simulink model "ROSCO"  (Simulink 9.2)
settings: Solver=VariableStepAuto  StartTime=0.0  StopTime=TMax  RelTol=1e-3
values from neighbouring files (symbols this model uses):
  OutList = [OutList    [runFAST.m]    (also in ROSCO2Matlab.m = [])
undefined symbols (not defined in the file or in its folder): cosd, DiscIntNeverNeededParam, F, Parameter, R, rpm2radps, simu, sind, strmatch
libraries: simulink x10
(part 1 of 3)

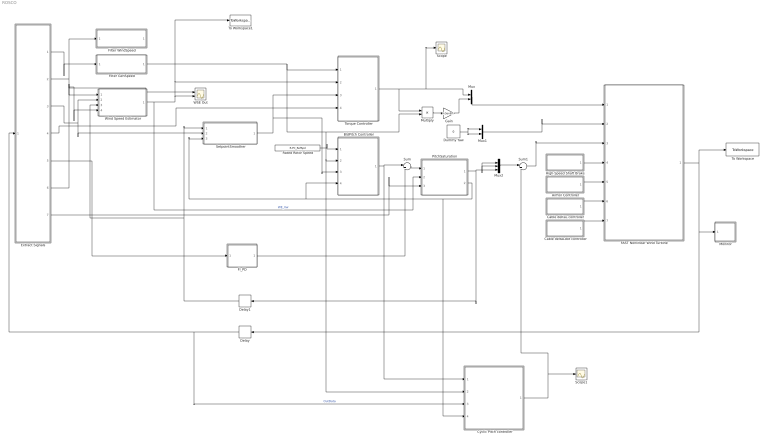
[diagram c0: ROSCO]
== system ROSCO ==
  AirFoil Controller : Subsystem
  BldPitch Controller : Subsystem
  Cable deltaL controller : Subsystem
  Cable deltaLdot controller : Subsystem
  Cyclic Pitch controller : Subsystem  TreatAsAtomicUnit=on
  Delay : Delay  Commented=through  DelayLength=1
  Delay1 : Delay  DelayLength=1
  Dummy Yaw : Constant  Value=0
  Extract Signals : Subsystem  TreatAsAtomicUnit=on
  FAST Nonlinear Wind Turbine : Subsystem
  Filter GenSpeed : Subsystem
  Filter WindSpeed : Subsystem
  Fl_PD : Subsystem
  Gain : Gain  Gain=R.GenEff
  High-Speed Shaft Brake : Subsystem
  Monitor : Subsystem  TreatAsAtomicUnit=on
  Multiply : Product
  Mux : Mux  Inputs=2
  Mux1 : Mux  Inputs=2
  Mux2 : Mux  Inputs=3
  PitchSaturation : Subsystem
  Rated Rotor Speed : Constant  Value=R.PC_RefSpd
  Scope : Scope
  Scope1 : Scope
  SetpointSmoother : Subsystem
  Sum : Sum  Inputs=|++
  Sum1 : Sum  Inputs=|++
  To Workspace : ToWorkspace  VariableName=FAST_Out  SaveFormat=Timeseries  SampleTime=-1
  To Workspace1 : ToWorkspace  VariableName=vhat  SaveFormat=Timeseries  SampleTime=-1
  Torque Controller : Subsystem
  WSE Out : Scope  NumInputPorts=2
  Wind Speed Estimator : Subsystem
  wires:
  FAST Nonlinear Wind Turbine/1(OutData) -> To Workspace/1, Delay/1, Monitor/1(OutData)
  Dummy Yaw/1 -> Mux1/2, Mux1/1
  Mux1/1 -> FAST Nonlinear Wind Turbine/2(Yaw Position (rad) and Rate (rad/s))
  Multiply/1 -> Gain/1
  Extract Signals/1(GenSpeed_rad/s) -> Filter GenSpeed/1(GenSpeed)
  Torque Controller/1(GenTq) -> Scope/1, Mux/1, Multiply/1
  Extract Signals/3(GenTq) -> Wind Speed Estimator/2(tau_g), SetpointSmoother/2(GenTq)
  SetpointSmoother/1(Del_Omega_g) -> BldPitch Controller/3(Del_omega_g), Torque Controller/3(Del_omega_g)
  Rated Rotor Speed/1 -> BldPitch Controller/1(omega_g,ref)
  Gain/1 -> Mux/2
  Extract Signals/2(RtVAvgxh) -> Wind Speed Estimator/4(HorWindV), WSE Out/1, Filter WindSpeed/1(WindSpeed)
  Wind Speed Estimator/1(v_hat) -> PitchSaturation/2(WE_Vw), WSE Out/2, Torque Controller/2(WindSpeedEst), To Workspace1/1  "WE_Vw"
  Delay/1 -> Cyclic Pitch controller/3(OutData), Extract Signals/1(OutData)  "OutData"
  Extract Signals/5(NcIMUTAys) -> Fl_PD/1(NacIMU)
  Fl_PD/1(Fl_Pitcom) -> Sum/2
  Extract Signals/4(BldPitch1) -> Torque Controller/4(BldPitch1)
  Sum/1 -> PitchSaturation/1(PitCom)
  PitchSaturation/1(PitCom_Sat) -> Delay1/1, Mux2/3, Mux2/1, Mux2/2
  PitchSaturation/2(PC_MinPitch) -> Cyclic Pitch controller/4(Min PItch (rad)), BldPitch Controller/4(Min Pitch), SetpointSmoother/3(MinPitch)
  BldPitch Controller/1(BldPitch) -> Cyclic Pitch controller/1(Coll. Pitch), Sum/1
  Extract Signals/6(RotSpeed (rad/s)) -> Wind Speed Estimator/1(omega_r)
  Delay1/1 -> SetpointSmoother/1(BldPitch1), Wind Speed Estimator/3(PitComT)
  Extract Signals/7(TwrFA Accel) -> PitchSaturation/3(TwrFA_Accel)
  Mux/1 -> FAST Nonlinear Wind Turbine/1(Gen. Torque (Nm) and Power (W))
  Filter GenSpeed/1(GenSpeedF) -> Torque Controller/1(GenSpeedF), Multiply/2, BldPitch Controller/2(GenSpeedF), Cyclic Pitch controller/2(Gen Speed)
  Cyclic Pitch controller/1(IPC Cmd (rad,3)) -> Scope1/1, Sum1/2
  Mux2/1 -> Sum1/1
  Sum1/1 -> FAST Nonlinear Wind Turbine/3(Blade Pitch Angles (rad))
  High-Speed Shaft Brake/1(Out1) -> FAST Nonlinear Wind Turbine/4(High-Speed Shaft Braking Fraction (-))
  AirFoil Controller/1(Out1) -> FAST Nonlinear Wind Turbine/5(AirFoil command (-))
  Cable deltaL controller/1(Out1) -> FAST Nonlinear Wind Turbine/6(Cable deltaL command (m))
  Cable deltaLdot controller/1(Out1) -> FAST Nonlinear Wind Turbine/7(Cable deltaLdot command (m/s))

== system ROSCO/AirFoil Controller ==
  Airfoil command : Constant  Value=zeros(1,3)'
  Out1 : Outport  VectorParamsAs1DForOutWhenUnconnected=on
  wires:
  Airfoil command/1 -> Out1/1

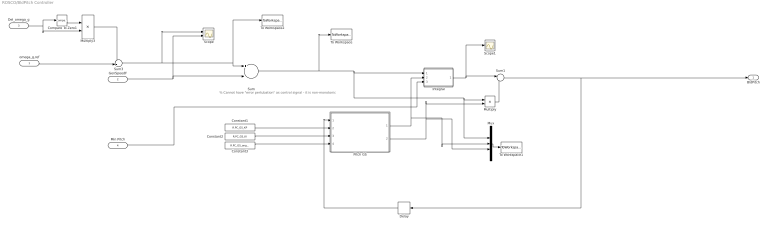
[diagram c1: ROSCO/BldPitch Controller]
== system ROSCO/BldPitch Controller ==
  note: % Cannot have "error pertubation" as control signal - it is non-monotonic
  omega_g,ref : Inport
  GenSpeedF : Inport  Port=2
  Del_omega_g : Inport  Port=3
  Min Pitch : Inport  Port=4
  Compare To Zero1 : simulink/Logic and Bit Operations/Compare To Zero  relop=<  OutDataTypeStr=boolean
  Constant1 : Constant  Value=R.PC_GS_KP
  Constant2 : Constant  Value=R.PC_GS_KI
  Constant3 : Constant  Value=R.PC_GS_angles
  Delay : Delay  DelayLength=1
  Integral : Subsystem
  Multiply : Product
  Multiply3 : Product
  Mux : Mux  Inputs=5
  Pitch GS : MATLAB Function  TreatAsAtomicUnit=on
  Scope : Scope  NumInputPorts=2
  Scope1 : Scope
  Sum : Sum  Inputs=+-
  Sum1 : Sum  Inputs=|++
  Sum3 : Sum  Inputs=-+|
  To Workspace : ToWorkspace  VariableName=SpdErr  SaveFormat=Timeseries  SampleTime=-1
  To Workspace1 : ToWorkspace  VariableName=PC_params  SaveFormat=Structure  SampleTime=-1
  To Workspace2 : ToWorkspace  VariableName=Omega_bg_ref  SaveFormat=Timeseries  SampleTime=-1
  BldPitch : Outport
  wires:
  Multiply/1 -> Sum1/2
  Integral/1(IntSpdErr) -> Scope1/1, Sum1/1
  Pitch GS/1(Ki) -> Mux/3, Integral/2(Gain)
  Pitch GS/2(Kp) -> Mux/4, Multiply/2
  Mux/1 -> To Workspace1/1
  Sum1/1 -> Delay/1, BldPitch/1
  Sum3/1 -> Scope/1, To Workspace2/1, Sum/1
  GenSpeedF/1 -> Scope/2, Sum/2
  Compare To Zero1/1 -> Multiply3/1
  Del_omega_g/1 -> Compare To Zero1/1, Multiply3/2
  Multiply3/1 -> Sum3/1
  omega_g,ref/1 -> Sum3/2
  Constant1/1 -> Pitch GS/2(Kp_pc)
  Constant2/1 -> Pitch GS/3(Ki_pc)
  Constant3/1 -> Pitch GS/4(PC_beta)
  Delay/1 -> Pitch GS/1(Beta)
  Min Pitch/1 -> Integral/3(Min Pitch)
  Sum/1 -> To Workspace/1, Mux/2, Multiply/1, Integral/1(SpeedErr)

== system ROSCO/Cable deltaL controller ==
  Cable deltaL command : Constant  Value=zeros(1,20)'
  Out1 : Outport  VectorParamsAs1DForOutWhenUnconnected=on
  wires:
  Cable deltaL command/1 -> Out1/1

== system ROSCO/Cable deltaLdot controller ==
  Cable deltaLdot command : Constant  Value=zeros(1,20)'
  Out1 : Outport  VectorParamsAs1DForOutWhenUnconnected=on
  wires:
  Cable deltaLdot command/1 -> Out1/1

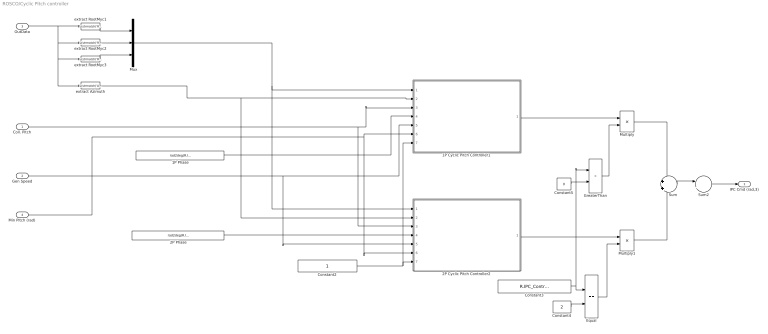
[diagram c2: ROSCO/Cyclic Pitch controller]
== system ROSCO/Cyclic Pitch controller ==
  Coll. Pitch : Inport
  Gen Speed : Inport  Port=2
  OutData : Inport  Port=3
  Min PItch (rad) : Inport  Port=4
  1P Cyclic Pitch Controller1 : Subsystem
  1P Phase : Constant  Value=rad2deg(R.IPC_aziOffset_1P)
  2P Cyclic Pitch Controller2 : Subsystem
  2P Phase : Constant  Value=rad2deg(R.IPC_aziOffset_2P)
  Constant2 : Constant
  Constant3 : Constant  Value=R.IPC_ControlMode
  Constant4 : Constant  Value=2
  Constant5 : Constant  Value=0
  Equal : RelationalOperator  Operator===  OutDataTypeStr=boolean  RndMeth=Simplest
  GreaterThan : RelationalOperator  Operator=>  OutDataTypeStr=boolean  RndMeth=Simplest
  Multiply : Product
  Multiply1 : Product
  Mux : Mux  Inputs=3
  Sum : Sum  Inputs=+|+
  Sum2 : Sum  Inputs=|++
  extract Azimuth : Fcn  Expr=u(strmatch('Azimuth',OutList))
  extract RootMyc1 : Fcn  Expr=u(strmatch('RootMyc1',OutList))
  extract RootMyc2 : Fcn  Expr=u(strmatch('RootMyc2',OutList))
  extract RootMyc3 : Fcn  Expr=u(strmatch('RootMyc3',OutList))
  IPC Cmd (rad,3) : Outport
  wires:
  1P Phase/1 -> 1P Cyclic Pitch Controller1/4(Phase (deg))
  Coll. Pitch/1 -> 2P Cyclic Pitch Controller2/3(Col. Pitch (rad)), 1P Cyclic Pitch Controller1/3(Col. Pitch (rad))
  Gen Speed/1 -> 2P Cyclic Pitch Controller2/5(Gen Speed (rpm)), 1P Cyclic Pitch Controller1/5(Gen Speed (rpm))
  1P Cyclic Pitch Controller1/1(IPC Cmd (rad,3)) -> Multiply/1
  extract RootMyc1/1 -> Mux/1
  extract RootMyc2/1 -> Mux/2
  extract RootMyc3/1 -> Mux/3
  Mux/1 -> 1P Cyclic Pitch Controller1/1(RootMyb), 2P Cyclic Pitch Controller2/1(RootMyb)
  extract Azimuth/1 -> 2P Cyclic Pitch Controller2/2(Azimuth (deg)), 1P Cyclic Pitch Controller1/2(Azimuth (deg))
  Min PItch (rad)/1 -> 2P Cyclic Pitch Controller2/6(Min Pitch (rad)), 1P Cyclic Pitch Controller1/6(Min Pitch (rad))
  2P Phase/1 -> 2P Cyclic Pitch Controller2/4(Phase (deg))
  2P Cyclic Pitch Controller2/1(IPC Cmd (rad,3)) -> Multiply1/1
  Multiply1/1 -> Sum/2
  Multiply/1 -> Sum/1
  OutData/1 -> extract Azimuth/1, extract RootMyc3/1, extract RootMyc2/1, extract RootMyc1/1
  Sum/1 -> Sum2/1
  Sum2/1 -> IPC Cmd (rad,3)/1
  Constant2/1 -> 1P Cyclic Pitch Controller1/7(Enable (-)), 2P Cyclic Pitch Controller2/7(Enable (-))
  Constant4/1 -> Equal/2
  Equal/1 -> Multiply1/2
  Constant3/1 -> GreaterThan/1, Equal/1
  Constant5/1 -> GreaterThan/2
  GreaterThan/1 -> Multiply/2

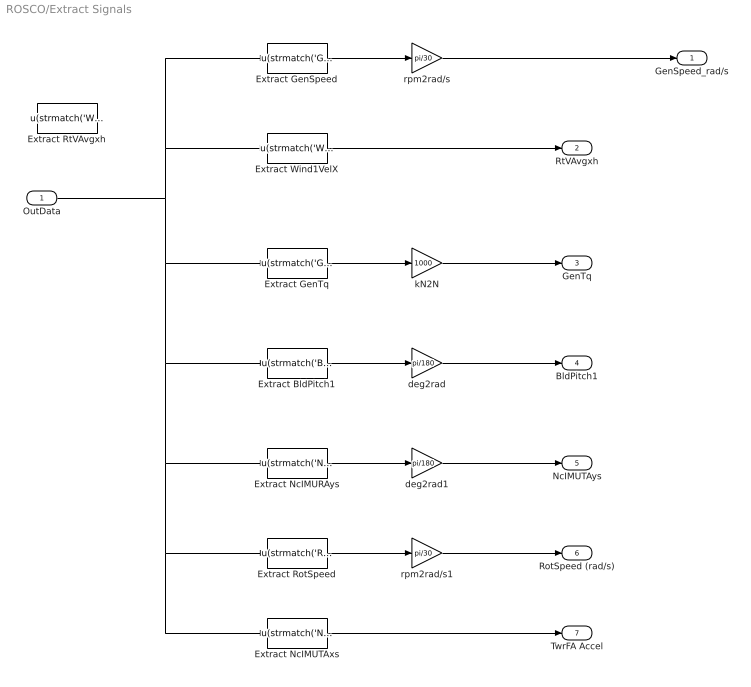
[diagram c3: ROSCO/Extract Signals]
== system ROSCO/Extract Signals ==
  OutData : Inport
  Extract BldPitch1 : Fcn  Expr=u(strmatch('BldPitch1',OutList))
  Extract GenSpeed : Fcn  Expr=u(strmatch('GenSpeed',OutList))
  Extract GenTq : Fcn  Expr=u(strmatch('GenTq',OutList))
  Extract NcIMURAys : Fcn  Expr=u(strmatch('NcIMURAys',OutList))
  Extract NcIMUTAxs : Fcn  Expr=u(strmatch('NcIMUTAxs',OutList))
  Extract RotSpeed : Fcn  Expr=u(strmatch('RotSpeed',OutList))
  Extract RtVAvgxh : Fcn  Commented=on  Expr=u(strmatch('Wind1VelX',OutList))
  Extract Wind1VelX : Fcn  Expr=u(strmatch('Wind1VelX',OutList))
  deg2rad : Gain  Gain=pi/180
  deg2rad1 : Gain  Gain=pi/180
  kN2N : Gain  Gain=1000
  rpm2rad/s : Gain  Gain=pi/30
  rpm2rad/s1 : Gain  Gain=pi/30
  GenSpeed_rad/s : Outport
  RtVAvgxh : Outport  Port=2
  GenTq : Outport  Port=3
  BldPitch1 : Outport  Port=4
  NcIMUTAys : Outport  Port=5
  RotSpeed (rad/s) : Outport  Port=6
  TwrFA Accel : Outport  Port=7
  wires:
  OutData/1 -> Extract Wind1VelX/1, Extract GenSpeed/1, Extract NcIMUTAxs/1, Extract RotSpeed/1, Extract NcIMURAys/1, Extract BldPitch1/1, Extract GenTq/1
  Extract Wind1VelX/1 -> RtVAvgxh/1
  Extract GenSpeed/1 -> rpm2rad/s/1
  Extract BldPitch1/1 -> deg2rad/1
  deg2rad/1 -> BldPitch1/1
  Extract GenTq/1 -> kN2N/1
  kN2N/1 -> GenTq/1
  Extract NcIMURAys/1 -> deg2rad1/1
  deg2rad1/1 -> NcIMUTAys/1
  Extract RotSpeed/1 -> rpm2rad/s1/1
  rpm2rad/s1/1 -> RotSpeed (rad/s)/1
  Extract NcIMUTAxs/1 -> TwrFA Accel/1
  rpm2rad/s/1 -> GenSpeed_rad/s/1

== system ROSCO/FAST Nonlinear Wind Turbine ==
  Gen. Torque (Nm) and Power (W) : Inport
  Yaw Position (rad) and Rate (rad/s) : Inport  Port=2
  Blade Pitch Angles (rad) : Inport  Port=3
  High-Speed Shaft Braking Fraction (-) : Inport  Port=4
  AirFoil command (-) : Inport  Port=5
  Cable deltaL command (m) : Inport  Port=6
  Cable deltaLdot command (m/s) : Inport  Port=7
  Mux1 : Mux  Inputs=7
  S-Function : S-Function  FunctionName=FAST_SFunc  Parameters=FAST_InputFileName, TMax, 43  SFunctionDeploymentMode=off  EnableBusSupport=off
  Signal Specification1 : SignalSpecification  OutDataTypeStr=double  Dimensions=2
  Signal Specification2 : SignalSpecification  OutDataTypeStr=double  Dimensions=2
  OutData : Outport  VectorParamsAs1DForOutWhenUnconnected=on
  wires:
  Gen. Torque (Nm) and Power (W)/1 -> Signal Specification1/1
  S-Function/1 -> OutData/1
  Mux1/1 -> S-Function/1
  Blade Pitch Angles (rad)/1 -> Mux1/3
  Yaw Position (rad) and Rate (rad/s)/1 -> Signal Specification2/1
  Signal Specification1/1 -> Mux1/1
  Signal Specification2/1 -> Mux1/2
  High-Speed Shaft Braking Fraction (-)/1 -> Mux1/4
  AirFoil command (-)/1 -> Mux1/5
  Cable deltaL command (m)/1 -> Mux1/6
  Cable deltaLdot command (m/s)/1 -> Mux1/7

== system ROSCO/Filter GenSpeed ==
  GenSpeed : Inport
  Discrete Filter : DiscreteFilter  Numerator=F.HSS.b  Denominator=F.HSS.a  InitialStates=R.VS_RefSpd/(sum(F.HSS.a(2:end))+1)
  Scope : Scope  NumInputPorts=2
  To Workspace2 : ToWorkspace  VariableName=Om_f  SaveFormat=Timeseries  SampleTime=-1
  GenSpeedF : Outport
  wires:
  Discrete Filter/1 -> Scope/2, To Workspace2/1, GenSpeedF/1
  GenSpeed/1 -> Scope/1, Discrete Filter/1

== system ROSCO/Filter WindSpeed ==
  WindSpeed : Inport
  Discrete Filter : DiscreteFilter  Numerator=F.Wind.b  Denominator=F.Wind.a  InitialStates=10
  To Workspace2 : ToWorkspace  VariableName=WindSpeedF  SaveFormat=Timeseries  SampleTime=-1
  WindSpeedF : Outport
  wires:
  Discrete Filter/1 -> WindSpeedF/1, To Workspace2/1
  WindSpeed/1 -> Discrete Filter/1

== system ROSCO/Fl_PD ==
  NacIMU : Inport
  Constant : Constant
  Enable : Gain  Gain=R.Fl_Mode
  Fl_HPF : DiscreteFilter  Numerator=F.F_Fl_HPF.b  Denominator=F.F_Fl_HPF.b
  Fl_LPF : DiscreteFilter  Numerator=F.F_Fl.b  Denominator=F.F_Fl.a
  Gain1 : Gain  Gain=-R.Fl_Kp
  Integral : Subsystem
  Scope : Scope
  Fl_Pitcom : Outport  VectorParamsAs1DForOutWhenUnconnected=on
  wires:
  Constant/1 -> Integral/2(Gain)
  NacIMU/1 -> Fl_LPF/1  "FA_AccR"
  Integral/1(Int x) -> Gain1/1
  Fl_HPF/1 -> Integral/1(x)  "FA_AccF"
  Gain1/1 -> Enable/1  "Fl_Pitcom"
  Enable/1 -> Scope/1, Fl_Pitcom/1  "Fl_Pitcom"
  Fl_LPF/1 -> Fl_HPF/1  "FA_AccF"

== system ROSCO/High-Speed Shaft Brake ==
  High-Speed Shaft Braking Fraction : Constant  Value=0
  Out1 : Outport  VectorParamsAs1DForOutWhenUnconnected=on
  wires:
  High-Speed Shaft Braking Fraction/1 -> Out1/1

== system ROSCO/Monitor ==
  OutData : Inport
  Extract BldPitch1 : Fcn  Expr=u(strmatch('BldPitch1',OutList))
  Extract GenTq : Fcn  Expr=u(strmatch('GenTq',OutList))
  Extract RotSpeed : Fcn  Expr=u(strmatch('RotSpeed',OutList))
  Scope : Scope  NumInputPorts=3
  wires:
  Extract BldPitch1/1 -> Scope/3
  OutData/1 -> Extract RotSpeed/1, Extract BldPitch1/1, Extract GenTq/1
  Extract RotSpeed/1 -> Scope/1
  Extract GenTq/1 -> Scope/2

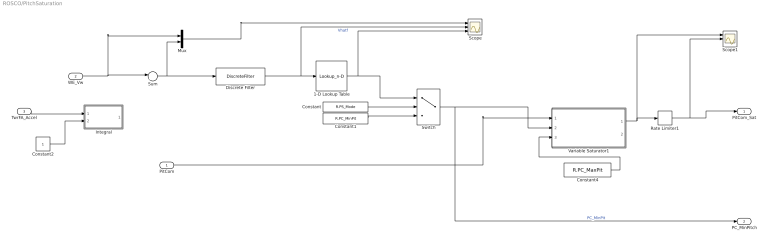
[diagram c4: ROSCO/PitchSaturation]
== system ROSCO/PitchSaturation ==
  PitCom : Inport
  WE_Vw : Inport  Port=2
  TwrFA_Accel : Inport  Port=3
  1-D Lookup Table : Lookup_n-D  NumberOfTableDimensions=1  BreakpointsForDimension1=R.PS_WindSpeeds  Table=R.PS_BldPitchMin  InternalRulePriority=Speed  RndMeth=Simplest
  Constant : Constant  Value=R.PS_Mode
  Constant1 : Constant  Value=R.PC_MinPit
  Constant2 : Constant
  Constant4 : Constant  Value=R.PC_MaxPit
  Discrete Filter : DiscreteFilter  Numerator=F.F_PS.b  Denominator=F.F_PS.a  InitialStates=R.WE_v0/(sum(F.F_PS.a(2:end))+1)
  Integral : Subsystem
  Mux : Mux  Inputs=2
  Rate Limiter1 : RateLimiter  RisingSlewLimit=R.PC_MaxRat  FallingSlewLimit=-R.PC_MaxRat  SampleTimeMode=inherited
  Scope : Scope  NumInputPorts=3
  Scope1 : Scope  NumInputPorts=3
  Sum : Sum  Inputs=|++
  Switch : Switch  Criteria=u2 > Threshold  Threshold=0.5
  Variable Saturator1 : MATLAB Function  TreatAsAtomicUnit=on
  PitCom_Sat : Outport  VectorParamsAs1DForOutWhenUnconnected=on
  PC_MinPitch : Outport  Port=2  VectorParamsAs1DForOutWhenUnconnected=on
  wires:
  1-D Lookup Table/1 -> Scope/3, Switch/1
  Constant/1 -> Switch/2
  Discrete Filter/1 -> Scope/2, 1-D Lookup Table/1  "Vhatf"
  Constant1/1 -> Switch/3
  Switch/1 -> PC_MinPitch/1, Variable Saturator1/2(lowerLimit)  "PC_MinPit"
  Constant4/1 -> Variable Saturator1/3(upperLimit)
  Variable Saturator1/1(pitchCommandOut) -> Scope1/1, Rate Limiter1/1
  Rate Limiter1/1 -> Scope1/2, PitCom_Sat/1
  PitCom/1 -> Variable Saturator1/1(pitchCommand)
  TwrFA_Accel/1 -> Integral/1(x)
  Constant2/1 -> Integral/2(Gain)
  WE_Vw/1 -> Mux/1, Sum/1
  Sum/1 -> Mux/2, Discrete Filter/1
  Mux/1 -> Scope/1

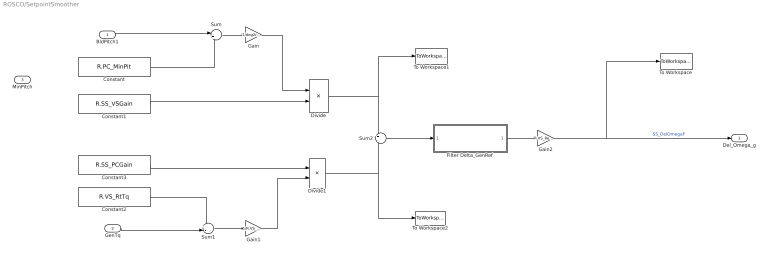
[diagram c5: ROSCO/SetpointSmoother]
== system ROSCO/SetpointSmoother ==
  BldPitch1 : Inport
  GenTq : Inport  Port=2
  MinPitch : Inport  Port=3
  Constant : Constant  Value=R.PC_MinPit
  Constant1 : Constant  Value=R.SS_VSGain
  Constant2 : Constant  Value=R.VS_RtTq
  Constant3 : Constant  Value=R.SS_PCGain
  Divide : Product  Inputs=**
  Divide1 : Product  Inputs=**
  Filter Delta_GenRef : Subsystem
  Gain : Gain  Gain=1/deg2rad(30)
  Gain1 : Gain  Gain=1/R.VS_RtTq
  Gain2 : Gain  Gain=R.VS_RefSpd
  Sum : Sum  Inputs=|+-
  Sum1 : Sum  Inputs=+-|
  Sum2 : Sum  Inputs=+|-
  To Workspace : ToWorkspace  VariableName=DelOmega  SaveFormat=Timeseries  SampleTime=-1
  To Workspace1 : ToWorkspace  VariableName=BldPitch_GB  SaveFormat=Timeseries  SampleTime=-1
  To Workspace2 : ToWorkspace  VariableName=Torque_GB  SaveFormat=Timeseries  SampleTime=-1
  Del_Omega_g : Outport
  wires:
  Divide1/1 -> Sum2/2, To Workspace2/1
  Divide/1 -> Sum2/1, To Workspace1/1
  Filter Delta_GenRef/1(GainBiasF) -> Gain2/1
  Constant3/1 -> Divide1/1
  Constant1/1 -> Divide/2
  Sum/1 -> Gain/1
  BldPitch1/1 -> Sum/1
  Sum2/1 -> Filter Delta_GenRef/1(GainBias)
  Constant2/1 -> Sum1/1
  Sum1/1 -> Gain1/1
  GenTq/1 -> Sum1/2
  Gain/1 -> Divide/1
  Gain1/1 -> Divide1/2
  Gain2/1 -> To Workspace/1, Del_Omega_g/1  "SS_DelOmegaF"
  Constant/1 -> Sum/2

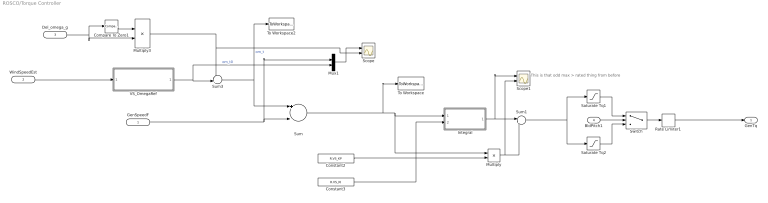
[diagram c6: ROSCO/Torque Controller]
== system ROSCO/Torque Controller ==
  note: This is that odd max > rated thing from before
  GenSpeedF : Inport
  WindSpeedEst : Inport  Port=2
  Del_omega_g : Inport  Port=3
  BldPitch1 : Inport  Port=4
  Compare To Zero1 : simulink/Logic and Bit Operations/Compare To Zero  relop=>  OutDataTypeStr=boolean
  Constant2 : Constant  Value=R.VS_KP
  Constant3 : Constant  Value=R.VS_KI
  Integral : Subsystem
  Multiply : Product
  Multiply3 : Product
  Mux1 : Mux  Inputs=2
  Rate Limiter1 : RateLimiter  RisingSlewLimit=R.VS_MaxRat  FallingSlewLimit=-R.VS_MaxRat  SampleTimeMode=inherited  InitialCondition=R.VS_RtTq
  Saturate Tq1 : Saturate  UpperLimit=R.VS_RtTq  LowerLimit=0
  Saturate Tq2 : Saturate  UpperLimit=R.VS_RtTq  LowerLimit=0
  Scope : Scope  NumInputPorts=2
  Scope1 : Scope  NumInputPorts=2
  Sum : Sum  Inputs=+-
  Sum1 : Sum  Inputs=|++
  Sum3 : Sum  Inputs=-+|
  Switch : Switch  Criteria=u2 > Threshold  Threshold=R.VS_Rgn3MP
  To Workspace : ToWorkspace  VariableName=VSdiff  SaveFormat=Timeseries  SampleTime=-1
  To Workspace2 : ToWorkspace  VariableName=Omega_tg_ref  SaveFormat=Timeseries  SampleTime=-1
  VS_OmegaRef : Subsystem
  GenTq : Outport
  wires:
  Multiply/1 -> Scope1/2, Sum1/2
  Integral/1(IntSpdErr) -> Scope1/1, Sum1/1
  Constant2/1 -> Multiply/2
  Constant3/1 -> Integral/2(Gain)
  VS_OmegaRef/1(VS_OmegaOpt) -> Mux1/2, Sum3/2  "om_t0"
  GenSpeedF/1 -> Mux1/1, Sum/2
  Sum3/1 -> To Workspace2/1, Sum/1  "om_t"
  Saturate Tq2/1 -> Switch/3
  Switch/1 -> Rate Limiter1/1
  Saturate Tq1/1 -> Switch/1
  BldPitch1/1 -> Switch/2
  Compare To Zero1/1 -> Multiply3/1
  Del_omega_g/1 -> Compare To Zero1/1, Multiply3/2
  Multiply3/1 -> Scope/2, Sum3/1
  Mux1/1 -> Scope/1
  Sum1/1 -> Saturate Tq2/1, Saturate Tq1/1
  Rate Limiter1/1 -> GenTq/1
  Sum/1 -> To Workspace/1, Integral/1(SpeedErr), Multiply/1
  WindSpeedEst/1 -> VS_OmegaRef/1(WindSpeedEst)

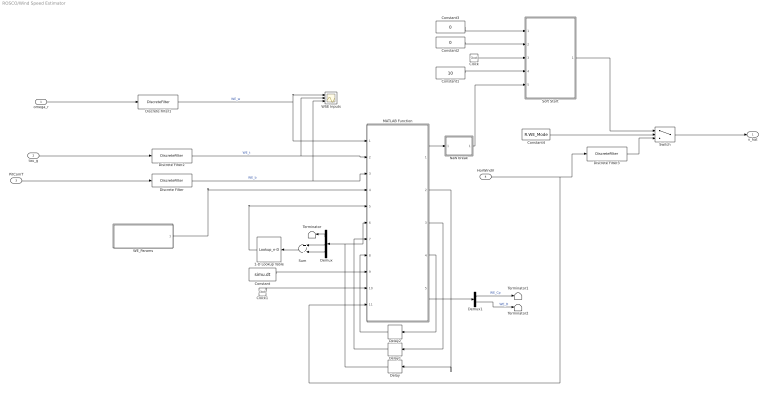
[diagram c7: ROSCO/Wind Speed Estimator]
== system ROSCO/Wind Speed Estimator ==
  omega_r : Inport
  tau_g : Inport  Port=2
  PitComT : Inport  Port=3
  HorWindV : Inport  Port=4
  1-D Lookup Table : Lookup_n-D  NumberOfTableDimensions=1  BreakpointsForDimension1=[-5:5]  Table=tanh([-5:5])  InternalRulePriority=Speed  RndMeth=Simplest
  Clock : Clock
  Clock1 : Clock
  Constant : Constant  Value=simu.dt
  Constant1 : Constant  Value=10
  Constant2 : Constant  Value=0
  Constant3 : Constant  Value=0
  Constant4 : Constant  Value=R.WE_Mode
  Delay : Delay  DelayLength=1  InitialCondition=[R.WE_GearboxRatio, 0, R.WE_v0]'
  Delay1 : Delay  DelayLength=1  InitialCondition=diag([0.1, 0.1, 1])^2
  Delay2 : Delay  DelayLength=1  InitialCondition=zeros(3,1)
  Demux : Demux  Outputs=3
  Demux1 : Demux  Outputs=2
  Discrete Filter : DiscreteFilter  Numerator=F.F_WSEBlPitch.b  Denominator=F.F_WSEBlPitch.a
  Discrete Filter1 : DiscreteFilter  Numerator=F.HSS.b  Denominator=F.HSS.a  InitialStates=R.VS_RefSpd/(sum(F.HSS.a(2:end))+1)/R.GBRatio
  Discrete Filter2 : DiscreteFilter  Numerator=F.F_GenTq.b  Denominator=F.F_GenTq.a  InitialStates=R.VS_RtTq/(sum(F.F_GenTq.a(2:end))+1)
  Discrete Filter3 : DiscreteFilter  Numerator=F.Wind.b  Denominator=F.Wind.a  InitialStates=10
  MATLAB Function : MATLAB Function  TreatAsAtomicUnit=on
  NaN break : MATLAB Function  TreatAsAtomicUnit=on
  Soft Start : MATLAB Function  TreatAsAtomicUnit=on
  Sum : Sum
  Switch : Switch  Criteria=u2 > Threshold  Threshold=0.5
  Terminator : Terminator
  Terminator1 : Terminator
  Terminator2 : Terminator
  WE_Params : Subsystem
  WSE Inputs : Scope  NumInputPorts=3
  v_hat : Outport
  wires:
  MATLAB Function/2(xh) -> Delay/1
  Delay/1 -> Demux/1, MATLAB Function/6("xh ")
  MATLAB Function/3(P) -> Delay1/1
  Delay1/1 -> MATLAB Function/7("P ")
  omega_r/1 -> Discrete Filter1/1
  tau_g/1 -> Discrete Filter2/1
  MATLAB Function/4(K) -> Delay2/1
  Delay2/1 -> MATLAB Function/8("K ")
  Constant/1 -> MATLAB Function/9(dt)
  Demux/2 -> Sum/1
  Demux/3 -> Sum/2
  Demux/1 -> Terminator/1
  Sum/1 -> 1-D Lookup Table/1
  1-D Lookup Table/1 -> MATLAB Function/5(A_op)
  WE_Params/1(WE_Params) -> MATLAB Function/4(WE_params)
  Clock/1 -> Soft Start/3(time)
  Constant1/1 -> Soft Start/4(generic)
  Constant2/1 -> Soft Start/2(endTime)
  Constant3/1 -> Soft Start/1(startTime)
  MATLAB Function/1(vh) -> NaN break/1(u)
  Discrete Filter/1 -> WSE Inputs/3, MATLAB Function/3(beta)  "WE_b"
  Discrete Filter1/1 -> MATLAB Function/1(omega_r), WSE Inputs/1  "WE_w"
  Discrete Filter2/1 -> MATLAB Function/2(tau_g), WSE Inputs/2  "WE_t"
  PitComT/1 -> Discrete Filter/1
  Soft Start/1(out) -> Switch/1
  Switch/1 -> v_hat/1
  HorWindV/1 -> MATLAB Function/11(HorWind), Discrete Filter3/1
  Constant4/1 -> Switch/2
  MATLAB Function/5(Debug) -> Demux1/1
  Demux1/1 -> Terminator1/1  "WE_Cp"
  Demux1/2 -> Terminator2/1  "WE_D"
  Clock1/1 -> MATLAB Function/10(t)
  Discrete Filter3/1 -> Switch/3
  NaN break/1(y) -> Soft Start/5(actual)

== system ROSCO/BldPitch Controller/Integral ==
  SpeedErr : Inport
  Gain : Inport  Port=2
  Min Pitch : Inport  Port=3
  Gain1 : Gain  Gain=simu.dt
  Maximum Pitch : Constant  Value=R.PC_MaxPit
  Minimum Pitch : Constant  Value=R.PC_MinPit
  Multiply : Product
  Saturate Integral Term : simulink/Discontinuities/Saturation Dynamic  OutMin=[]  OutMax=[]  OutDataTypeStr=Inherit: Same as second input  OutDataType=fixdt(1, 16)  OutScaling=2^-10  RndMeth=Nearest  DoSatur=off
  Sum : Sum  Inputs=|++
  Unit Delay : UnitDelay  SampleTime=-1
  IntSpdErr : Outport
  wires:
  Maximum Pitch/1 -> Saturate Integral Term/1
  Unit Delay/1 -> Sum/2
  Sum/1 -> Saturate Integral Term/2
  SpeedErr/1 -> Gain1/1
  Gain/1 -> Multiply/2
  Saturate Integral Term/1 -> IntSpdErr/1, Unit Delay/1
  Gain1/1 -> Multiply/1
  Multiply/1 -> Sum/1
  Min Pitch/1 -> Saturate Integral Term/3

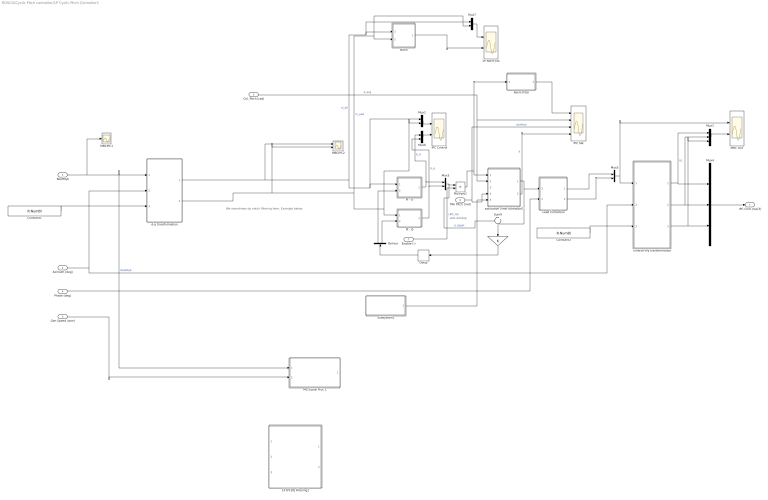
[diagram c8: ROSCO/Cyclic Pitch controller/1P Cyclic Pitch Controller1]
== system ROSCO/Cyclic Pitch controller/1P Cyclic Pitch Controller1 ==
  note: We sometimes do notch filtering here. Example below.
  note: k
  note: anti-windup
  RootMyb : Inport
  Azimuth (deg) : Inport  Port=2
  Col. Pitch (rad) : Inport  Port=3
  Phase (deg) : Inport  Port=4
  Gen Speed (rpm) : Inport  Port=5
  Min Pitch (rad) : Inport  Port=6
  Enable (-) : Inport  Port=7
  " " : Gain
  1P IPCDQ Filtering1 : Subsystem  Commented=on
  1P Norm Est : Scope  NumInputPorts=2
  Constant1 : Constant  Value=R.NumBl
  Constant2 : Constant  Value=R.NumBl
  Delay : Delay  DelayLength=1
  Demux : Demux  Outputs=2
  IPC Control : Scope  NumInputPorts=2
  IPC Sat : Scope  NumInputPorts=4
  Lead Correction : MATLAB Function  TreatAsAtomicUnit=on
  M0 Signal Proc.1 : Subsystem  Commented=on
  MBC Out : Scope  NumInputPorts=2
  MBCIPC1 : Scope
  MBCIPC2 : Scope  NumInputPorts=2
  Multiply1 : Product
  Mux1 : Mux  Inputs=3
  Mux{2..3,5..7} (5 alike) : Mux  Inputs=2
  Mux4 : Mux  Inputs=3
  Norm : Subsystem  Commented=on
  Norm Pitch : Subsystem  Commented=on
  PI - D : Subsystem  TreatAsAtomicUnit=on  SystemSampleTime=simu.dt
  PI - Q : Subsystem  TreatAsAtomicUnit=on  SystemSampleTime=simu.dt
  Subsystem1 : Subsystem
  Sum9 : Sum  Inputs=-|+
  d-q transformation : MATLAB Function  TreatAsAtomicUnit=on
  inverse d-q transformation : MATLAB Function  TreatAsAtomicUnit=on
  saturation (limit schedule)1 : MATLAB Function  TreatAsAtomicUnit=on
  IPC Cmd (rad,3) : Outport
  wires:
  Col. Pitch (rad)/1 -> saturation (limit schedule)1/2(b_avg), IPC Sat/2  "b_avg"
  saturation (limit schedule)1/1(bdq) -> Sum9/2, Lead Correction/1(bdq)
  Gen Speed (rpm)/1 -> M0 Signal Proc.1/2(GenSpeed)
  d-q transformation/1(M_tilt) -> Mux2/1, PI - D/1(Md), Mux7/1, Norm/1(In1), MBCIPC2/1  "m_tilt"
  Mux5/1 -> MBC Out/1, inverse d-q transformation/1(bdq)
  inverse d-q transformation/3(b3) -> Mux1/3, Mux4/3
  Phase (deg)/1 -> Lead Correction/2(psi_o)
  PI - Q/1(Theta_yaw) -> Mux6/2, Mux3/2  "b_q"
  PI - D/1(Theta_tilt) -> Mux3/1, Mux6/1  "b_d"
  Demux/1 -> PI - D/2(Anti-windup)
  inverse d-q transformation/1(b1) -> Mux1/1, Mux4/1  "b1"
  Demux/2 -> PI - Q/2(Anti-windup)
  inverse d-q transformation/2(b2) -> Mux1/2, Mux4/2
  Mux4/1 -> IPC Cmd (rad,3)/1
  Delay/1 -> Demux/1
  " "/1 -> Delay/1
  RootMyb/1 -> M0 Signal Proc.1/1("My1,2, 3"), d-q transformation/1(RootMyb), MBCIPC1/1  "RootMyb"
  Sum9/1 -> " "/1
  Azimuth (deg)/1 -> d-q transformation/2(Az), inverse d-q transformation/2(Az)
  Lead Correction/1(b_cos) -> Mux5/1
  Lead Correction/2(b_sin) -> Mux5/2
  saturation (limit schedule)1/2(k) -> IPC Sat/4
  Constant1/1 -> d-q transformation/3(NumBl)
  Constant2/1 -> inverse d-q transformation/3(NumBl)
  d-q transformation/2(M_yaw) -> Mux2/2, PI - Q/1(Mq), Mux7/2, Norm/2(In2), MBCIPC2/2  "m_yaw"
  Mux1/1 -> MBC Out/2
  Mux6/1 -> IPC Control/2
  Mux2/1 -> IPC Control/1
  Mux7/1 -> 1P Norm Est/1
  Norm/1(Out1) -> 1P Norm Est/2
  Min Pitch (rad)/1 -> IPC Sat/3, saturation (limit schedule)1/4(minPitch)  "minPitch"
  Norm Pitch/1(Out1) -> IPC Sat/1
  Enable (-)/1 -> Multiply1/2  "cIPC_GS"
  Subsystem1/1(IPC Sat Params) -> saturation (limit schedule)1/5(Params)
  Mux3/1 -> Sum9/1, Multiply1/1  "b_dqsat"
  Multiply1/1 -> Norm Pitch/1(b_dqsat), saturation (limit schedule)1/1(bdq_unsat)
  ? -> 1P IPCDQ Filtering1/2(My)  "m_yaw"

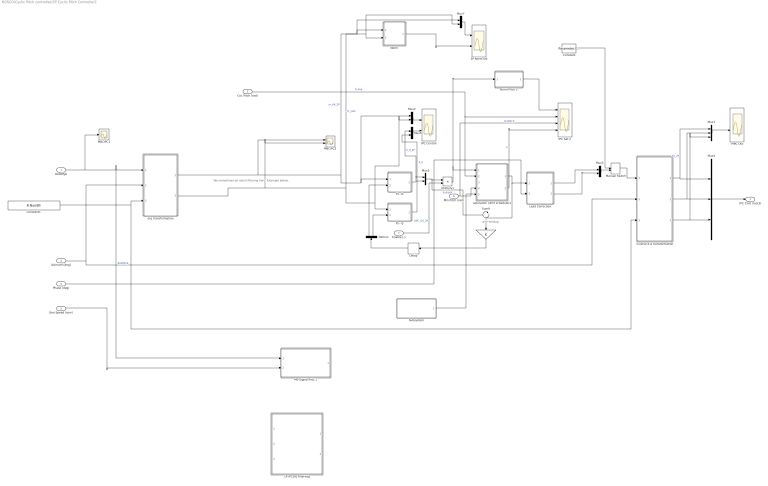
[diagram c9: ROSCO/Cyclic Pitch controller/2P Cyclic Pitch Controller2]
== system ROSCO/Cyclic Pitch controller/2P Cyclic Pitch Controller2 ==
  note: We sometimes do notch filtering here. Example below.
  note: anti-windup
  note: k
  RootMyb : Inport
  Azimuth (deg) : Inport  Port=2
  Col. Pitch (rad) : Inport  Port=3
  Phase (deg) : Inport  Port=4
  Gen Speed (rpm) : Inport  Port=5
  Min Pitch (rad) : Inport  Port=6
  Enable (-) : Inport  Port=7
  " " : Gain
  1P IPCDQ Filtering1 : Subsystem  Commented=on
  2P Norm Est : Scope  NumInputPorts=2
  Constant : Constant  Commented=on  Value=Parameter.Control.cIPC.OL_2P.amp * [cosd(Parameter.Control.cIPC.OL_2P.phase), sind(Parameter.Control.cIPC.OL_2P.phase)]
  Constant1 : Constant  Value=R.NumBl
  Delay : Delay  DelayLength=1
  Demux : Demux  Outputs=2
  IPC Control : Scope  NumInputPorts=2
  IPC Sat 2 : Scope  NumInputPorts=4
  Lead Correction : MATLAB Function  TreatAsAtomicUnit=on
  M0 Signal Proc.1 : Subsystem  Commented=on
  MBC Out : Scope  NumInputPorts=2
  MBCIPC1 : Scope
  MBCIPC2 : Scope  NumInputPorts=2
  Manual Switch : ManualSwitch  CurrentSetting=0
  Multiply1 : Product
  Mux1 : Mux  Inputs=3
  Mux{2..3,5..7} (5 alike) : Mux  Inputs=2
  Mux4 : Mux  Inputs=3
  Norm : Subsystem  Commented=on
  Norm Pitch 2 : Subsystem  Commented=on
  PI - D : Subsystem  TreatAsAtomicUnit=on  SystemSampleTime=simu.dt
  PI - Q : Subsystem  TreatAsAtomicUnit=on  SystemSampleTime=simu.dt
  Subsystem : Subsystem
  Sum9 : Sum  Inputs=-|+
  d-q transformation : MATLAB Function  TreatAsAtomicUnit=on
  inverse d-q transformation : MATLAB Function  TreatAsAtomicUnit=on
  saturation (limit schedule)1 : MATLAB Function  TreatAsAtomicUnit=on
  IPC Cmd (rad,3) : Outport
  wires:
  Enable (-)/1 -> Multiply1/2  "cIPC_GS_2P"
  Norm Pitch 2/1(Out1) -> IPC Sat 2/1
  Min Pitch (rad)/1 -> saturation (limit schedule)1/4(minPitch), IPC Sat 2/3  "minPitch"
  Norm/1(Out1) -> 2P Norm Est/2
  Mux7/1 -> 2P Norm Est/1
  Mux2/1 -> IPC Control/1
  Mux6/1 -> IPC Control/2
  Mux1/1 -> MBC Out/2
  d-q transformation/2(M_yaw) -> PI - Q/1(Mq), Mux2/2, Norm/2(In2), Mux7/2, MBCIPC2/2  "m_yaw"
  Constant1/1 -> inverse d-q transformation/3(NumBl), d-q transformation/3(NumBl)
  saturation (limit schedule)1/2(k) -> IPC Sat 2/4
  Lead Correction/2(b_sin) -> Mux5/2
  Lead Correction/1(b_cos) -> Mux5/1
  Azimuth (deg)/1 -> inverse d-q transformation/2(Az), d-q transformation/2(Az)
  Sum9/1 -> " "/1
  RootMyb/1 -> MBCIPC1/1, M0 Signal Proc.1/1("My1,2, 3"), d-q transformation/1(RootMyb)  "RootMyb"
  " "/1 -> Delay/1
  Delay/1 -> Demux/1
  Mux4/1 -> IPC Cmd (rad,3)/1
  inverse d-q transformation/2(b2) -> Mux4/2, Mux1/2
  Demux/2 -> PI - Q/2(Anti-windup)
  inverse d-q transformation/1(b1) -> Mux4/1, Mux1/1  "b1_2P"
  Demux/1 -> PI - D/2(Anti-windup)
  PI - D/1(Theta_tilt) -> Mux6/1, Mux3/1  "b_d_2P"
  PI - Q/1(Theta_yaw) -> Mux6/2, Mux3/2  "b_q"
  Phase (deg)/1 -> Lead Correction/2(psi_o)
  inverse d-q transformation/3(b3) -> Mux4/3, Mux1/3
  d-q transformation/1(M_tilt) -> PI - D/1(Md), Mux2/1, Norm/1(In1), Mux7/1, MBCIPC2/1  "m_tilt_2P"
  Gen Speed (rpm)/1 -> M0 Signal Proc.1/2(GenSpeed)
  saturation (limit schedule)1/1(bdq) -> Lead Correction/1(bdq), Sum9/2
  Col. Pitch (rad)/1 -> IPC Sat 2/2, saturation (limit schedule)1/2(b_avg)  "b_avg"
  Subsystem/1(IPC Sat Params) -> saturation (limit schedule)1/5(Params)
  Mux3/1 -> Sum9/1, Multiply1/1  "b_dqsat"
  Multiply1/1 -> Norm Pitch 2/1(b_dqsat), saturation (limit schedule)1/1(bdq_unsat)
  Mux5/1 -> Manual Switch/2
  Manual Switch/1 -> inverse d-q transformation/1(bdq)
  Constant/1 -> Manual Switch/1

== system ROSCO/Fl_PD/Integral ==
  x : Inport
  Gain : Inport  Port=2
  Gain1 : Gain  Gain=simu.dt
  Maximum Pitch : Constant  Value=100
  Minimum Pitch : Constant  Value=-100
  Multiply : Product
  Saturate Integral Term : simulink/Discontinuities/Saturation Dynamic  OutMin=[]  OutMax=[]  OutDataTypeStr=Inherit: Same as second input  OutDataType=fixdt(1, 16)  OutScaling=2^-10  RndMeth=Nearest  DoSatur=off
  Scope : Scope  NumInputPorts=2
  Sum : Sum  Inputs=|++
  Unit Delay : UnitDelay  SampleTime=-1
  Int x : Outport
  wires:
  Maximum Pitch/1 -> Saturate Integral Term/1
  Unit Delay/1 -> Sum/2
  Minimum Pitch/1 -> Saturate Integral Term/3
  Sum/1 -> Saturate Integral Term/2
  x/1 -> Scope/1, Gain1/1
  Gain/1 -> Multiply/2
  Saturate Integral Term/1 -> Scope/2, Int x/1, Unit Delay/1
  Gain1/1 -> Multiply/1
  Multiply/1 -> Sum/1

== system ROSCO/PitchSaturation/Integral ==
  x : Inport
  Gain : Inport  Port=2
  Gain1 : Gain  Gain=simu.dt
  Maximum Pitch : Constant  Value=100
  Minimum Pitch : Constant  Value=-100
  Multiply : Product
  Saturate Integral Term : simulink/Discontinuities/Saturation Dynamic  OutMin=[]  OutMax=[]  OutDataTypeStr=Inherit: Same as second input  OutDataType=fixdt(1, 16)  OutScaling=2^-10  RndMeth=Nearest  DoSatur=off
  Scope : Scope  NumInputPorts=2
  Sum : Sum  Inputs=|++
  Unit Delay : UnitDelay  SampleTime=-1
  Int x : Outport
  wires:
  Maximum Pitch/1 -> Saturate Integral Term/1
  Unit Delay/1 -> Sum/2
  Minimum Pitch/1 -> Saturate Integral Term/3
  Sum/1 -> Saturate Integral Term/2
  x/1 -> Scope/1, Gain1/1
  Gain/1 -> Multiply/2
  Saturate Integral Term/1 -> Scope/2, Int x/1, Unit Delay/1
  Gain1/1 -> Multiply/1
  Multiply/1 -> Sum/1

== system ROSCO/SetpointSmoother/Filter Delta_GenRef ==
  GainBias : Inport
  Discrete Filter : DiscreteFilter  Numerator=F.F_SS.b  Denominator=F.F_SS.a
  GainBiasF : Outport
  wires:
  Discrete Filter/1 -> GainBiasF/1
  GainBias/1 -> Discrete Filter/1

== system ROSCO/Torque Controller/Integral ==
  SpeedErr : Inport
  Gain : Inport  Port=2
  Gain1 : Gain  Gain=simu.dt
  Maximum Torque : Constant  Value=R.VS_RtTq
  Minimum Torque : Constant  Value=0
  Multiply : Product
  Saturate Integral Term : simulink/Discontinuities/Saturation Dynamic  OutMin=[]  OutMax=[]  OutDataTypeStr=Inherit: Same as second input  OutDataType=fixdt(1, 16)  OutScaling=2^-10  RndMeth=Nearest  DoSatur=off
  Sum : Sum  Inputs=|++
  Unit Delay : UnitDelay  InitialCondition=R.VS_RtTq  SampleTime=-1
  IntSpdErr : Outport
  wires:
  Maximum Torque/1 -> Saturate Integral Term/1
  Unit Delay/1 -> Sum/2
  Minimum Torque/1 -> Saturate Integral Term/3
  Sum/1 -> Saturate Integral Term/2
  SpeedErr/1 -> Gain1/1
  Gain/1 -> Multiply/2
  Saturate Integral Term/1 -> IntSpdErr/1, Unit Delay/1
  Gain1/1 -> Multiply/1
  Multiply/1 -> Sum/1

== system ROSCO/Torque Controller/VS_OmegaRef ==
  WindSpeedEst : Inport
  Omega_opt : Subsystem
  Reference TSR : Constant  Value=R.VS_TSRopt
  Saturation : Saturate  UpperLimit=R.PC_RefSpd  LowerLimit=R.VS_MinOMSpd
  To Workspace1 : ToWorkspace  VariableName=Om_opt  SaveFormat=Timeseries  SampleTime=-1
  VS_OmegaOpt : Outport
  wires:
  WindSpeedEst/1 -> Omega_opt/2(Wind Speed)
  Omega_opt/1(Omega_opt) -> Saturation/1
  Reference TSR/1 -> Omega_opt/1(TSR_opt)
  Saturation/1 -> VS_OmegaOpt/1, To Workspace1/1

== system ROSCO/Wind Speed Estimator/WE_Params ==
  Constant1 : Constant  Value=R.WE_Jtot
  Constant2 : Constant  Value=R.WE_RhoAir
  Constant3 : Constant  Value=R.WE_BladeRadius
  Constant4 : Constant  Value=R.WE_GearboxRatio
  Mux : Mux
  WE_Params : Outport  VectorParamsAs1DForOutWhenUnconnected=on
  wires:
  Constant2/1 -> Mux/2
  Mux/1 -> WE_Params/1
  Constant4/1 -> Mux/4
  Constant1/1 -> Mux/1
  Constant3/1 -> Mux/3

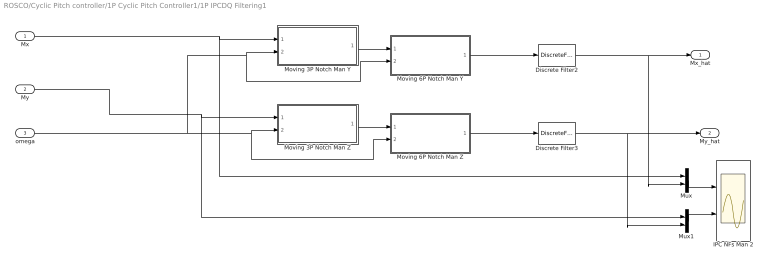
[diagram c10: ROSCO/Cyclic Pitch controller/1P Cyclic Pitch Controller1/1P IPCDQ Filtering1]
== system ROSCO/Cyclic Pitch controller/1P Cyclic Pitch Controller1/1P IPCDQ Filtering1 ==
  Mx : Inport
  My : Inport  Port=2
  omega : Inport  Port=3
  Discrete Filter2 : DiscreteFilter  Numerator=Parameter.Control.cIPC.IPCDQ_LPF.Numerator{1}  Denominator=Parameter.Control.cIPC.IPCDQ_LPF.Denominator{1}  SampleTime=Parameter.Control.DT
  Discrete Filter3 : DiscreteFilter  Numerator=Parameter.Control.cIPC.IPCDQ_LPF.Numerator{1}  Denominator=Parameter.Control.cIPC.IPCDQ_LPF.Denominator{1}  SampleTime=Parameter.Control.DT
  IPC NFs Man 2 : Scope  NumInputPorts=2
  Moving 3P Notch Man Y : Subsystem
  Moving 3P Notch Man Z : Subsystem
  Moving 6P Notch Man Y : Subsystem
  Moving 6P Notch Man Z : Subsystem
  Mux : Mux  Inputs=2
  Mux1 : Mux  Inputs=2
  Mx_hat : Outport
  My_hat : Outport  Port=2
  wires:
  omega/1 -> Moving 6P Notch Man Y/2(GenSpeedIN), Moving 3P Notch Man Y/2(GenSpeedIN), Moving 6P Notch Man Z/2(GenSpeedIN), Moving 3P Notch Man Z/2(GenSpeedIN)
  Mx/1 -> Mux/1, Moving 3P Notch Man Y/1(Input)
  My/1 -> Mux1/1, Moving 3P Notch Man Z/1(Input)
  Moving 6P Notch Man Z/1(Output) -> Discrete Filter3/1
  Moving 6P Notch Man Y/1(Output) -> Discrete Filter2/1
  Moving 3P Notch Man Y/1(Output) -> Moving 6P Notch Man Y/1(Input)
  Moving 3P Notch Man Z/1(Output) -> Moving 6P Notch Man Z/1(Input)
  Mux1/1 -> IPC NFs Man 2/2
  Mux/1 -> IPC NFs Man 2/1
  Discrete Filter3/1 -> Mux1/2, My_hat/1
  Discrete Filter2/1 -> Mux/2, Mx_hat/1

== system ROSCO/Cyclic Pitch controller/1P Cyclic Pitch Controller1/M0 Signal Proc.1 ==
  "My1,2, 3" : Inport
  GenSpeed : Inport  Port=2
  Add : Sum  Inputs=+++
  Demux1 : Demux  Outputs=3
  Discrete Filter : DiscreteFilter  Numerator=Parameter.Control.cIPC.PSM0_LPF.Numerator{1}  Denominator=Parameter.Control.cIPC.PSM0_LPF.Denominator{1}  a0EqualsOne=on
  Gain : Gain  Gain=1/3
  Moving 1P Notch Man : Subsystem
  Moving 3P Notch Man : Subsystem
  Mux : Mux  Inputs=2
  Scope : Scope  NumInputPorts=2
  M0 : Outport
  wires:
  Demux1/1 -> Add/1
  Demux1/2 -> Add/2
  Add/1 -> Gain/1
  "My1,2, 3"/1 -> Demux1/1
  GenSpeed/1 -> Moving 3P Notch Man/2(GenSpeedIN), Moving 1P Notch Man/2(GenSpeedIN)
  Demux1/3 -> Add/3
  Moving 1P Notch Man/1(Output) -> Moving 3P Notch Man/1(Input)
  Mux/1 -> Scope/2
  Gain/1 -> Scope/1, Moving 1P Notch Man/1(Input)
  Moving 3P Notch Man/1(Output) -> Discrete Filter/1
  Discrete Filter/1 -> Mux/1, M0/1

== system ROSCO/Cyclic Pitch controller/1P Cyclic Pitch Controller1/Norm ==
  In1 : Inport
  In2 : Inport  Port=2
  Add : Sum
  Discrete Filter1 : DiscreteFilter  Numerator=Parameter.Control.cIPC.IPCDQ_LPF.num{1}  Denominator=Parameter.Control.cIPC.IPCDQ_LPF.den{1}  SampleTime=Parameter.Control.DT
  Product : Product
  Product1 : Product
  Sqrt : Sqrt
  Out1 : Outport
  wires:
  Product/1 -> Add/1
  Product1/1 -> Add/2
  Sqrt/1 -> Discrete Filter1/1
  Add/1 -> Sqrt/1
  In2/1 -> Product1/1, Product1/2
  In1/1 -> Product/1, Product/2
  Discrete Filter1/1 -> Out1/1

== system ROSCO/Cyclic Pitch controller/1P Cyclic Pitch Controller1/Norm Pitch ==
  b_dqsat : Inport
  Demux1 : Demux  Outputs=2
  Sqrt : Sqrt
  Square : Math  Operator=square
  Square1 : Math  Operator=square
  Sum : Sum
  Out1 : Outport
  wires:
  Demux1/1 -> Square/1
  Square1/1 -> Sum/2
  b_dqsat/1 -> Demux1/1
  Sum/1 -> Sqrt/1
  Demux1/2 -> Square1/1
  Square/1 -> Sum/1
  Sqrt/1 -> Out1/1

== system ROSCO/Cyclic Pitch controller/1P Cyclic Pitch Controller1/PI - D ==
  Md : Inport
  Anti-windup : Inport  Port=2
  Discrete Derivative : simulink/Discrete/Discrete Derivative  gainval=1.0  ICPrevScaledInput=0.0  OutMin=[]  OutMax=[]  OutDataType=fixdt(1, 16)  OutScaling=2^-10  DoSatur=off
  Discrete Filter1 : DiscreteFilter  Commented=through  Numerator=Parameter.Control.cIPC.IPCDQ_LPF.num{1}  Denominator=Parameter.Control.cIPC.IPCDQ_LPF.den{1}  SampleTime=Parameter.Control.DT
  Integrator : DiscreteIntegrator  IntegratorMethod=Integration: Backward Euler  gainval=1  SampleTime=simu.dt  UpperSaturationLimit=1.570796/(.008068634/9.5492966)/(1./(1.+pi/2/.109997))  LowerSaturationLimit=0  ICPrevOutput=DiscIntNeverNeededParam  ICPrevScaledInput=DiscIntNeverNeededParam
  Kd : Gain  Gain=0
  Ki : Gain  Gain=R.IPC_KI_2P
  Kp : Gain  Gain=R.IPC_KP_1P
  Scope : Scope  NumInputPorts=2
  Sum3 : Sum  Inputs=+++
  Sum8 : Sum  Inputs=|++
  Theta_tilt : Outport
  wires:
  Ki/1 -> Sum8/1
  Sum3/1 -> Scope/1, Theta_tilt/1
  Md/1 -> Ki/1, Kp/1, Discrete Filter1/1
  Anti-windup/1 -> Scope/2, Sum8/2
  Sum8/1 -> Integrator/1
  Kd/1 -> Discrete Derivative/1
  Kp/1 -> Sum3/2
  Discrete Derivative/1 -> Sum3/1
  Integrator/1 -> Sum3/3
  Discrete Filter1/1 -> Kd/1

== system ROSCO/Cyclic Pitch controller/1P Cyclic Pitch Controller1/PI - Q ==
  Mq : Inport
  Anti-windup : Inport  Port=2
  Discrete Derivative : simulink/Discrete/Discrete Derivative  gainval=1.0  ICPrevScaledInput=0.0  OutMin=[]  OutMax=[]  OutDataType=fixdt(1, 16)  OutScaling=2^-10  DoSatur=off
  Discrete Filter1 : DiscreteFilter  Commented=through  Numerator=Parameter.Control.cIPC.IPCDQ_LPF.num{1}  Denominator=Parameter.Control.cIPC.IPCDQ_LPF.den{1}  SampleTime=Parameter.Control.DT
  Integrator1 : DiscreteIntegrator  IntegratorMethod=Integration: Backward Euler  gainval=1  SampleTime=simu.dt  UpperSaturationLimit=1.570796/(.008068634/9.5492966)/(1./(1.+pi/2/.109997))  LowerSaturationLimit=0  ICPrevOutput=DiscIntNeverNeededParam  ICPrevScaledInput=DiscIntNeverNeededParam
  Kd : Gain  Gain=0
  Ki : Gain  Gain=R.IPC_KI_1P
  Kp : Gain  Gain=R.IPC_KP_1P
  Sum10 : Sum  Inputs=|++
  Sum3 : Sum  Inputs=+++
  Theta_yaw : Outport
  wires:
  Sum3/1 -> Theta_yaw/1
  Sum10/1 -> Integrator1/1
  Anti-windup/1 -> Sum10/2
  Integrator1/1 -> Sum3/3
  Ki/1 -> Sum10/1
  Kp/1 -> Sum3/2
  Mq/1 -> Discrete Filter1/1, Kp/1, Ki/1
  Kd/1 -> Discrete Derivative/1
  Discrete Derivative/1 -> Sum3/1
  Discrete Filter1/1 -> Kd/1

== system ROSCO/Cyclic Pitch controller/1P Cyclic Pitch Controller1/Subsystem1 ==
  Constant3 : Constant  Value=2
  Constant4 : Constant  Value=0
  Constant5 : Constant  Value=0
  Mux : Mux  Inputs=3
  IPC Sat Params : Outport
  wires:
  Constant3/1 -> Mux/1
  Constant4/1 -> Mux/2
  Constant5/1 -> Mux/3
  Mux/1 -> IPC Sat Params/1

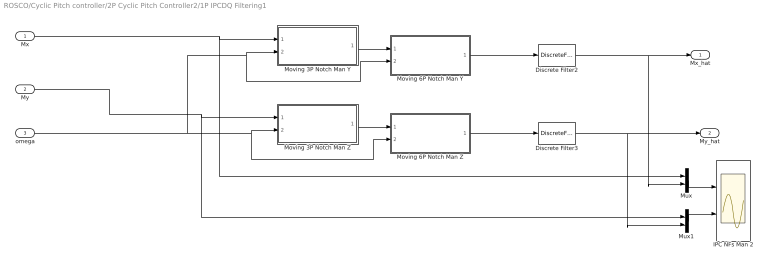
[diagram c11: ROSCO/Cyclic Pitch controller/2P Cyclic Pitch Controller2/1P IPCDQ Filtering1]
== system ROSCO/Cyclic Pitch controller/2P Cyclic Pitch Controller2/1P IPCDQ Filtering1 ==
  Mx : Inport
  My : Inport  Port=2
  omega : Inport  Port=3
  Discrete Filter2 : DiscreteFilter  Numerator=Parameter.Control.cIPC.IPCDQ_LPF.Numerator{1}  Denominator=Parameter.Control.cIPC.IPCDQ_LPF.Denominator{1}  SampleTime=Parameter.Control.DT
  Discrete Filter3 : DiscreteFilter  Numerator=Parameter.Control.cIPC.IPCDQ_LPF.Numerator{1}  Denominator=Parameter.Control.cIPC.IPCDQ_LPF.Denominator{1}  SampleTime=Parameter.Control.DT
  IPC NFs Man 2 : Scope  NumInputPorts=2
  Moving 3P Notch Man Y : Subsystem
  Moving 3P Notch Man Z : Subsystem
  Moving 6P Notch Man Y : Subsystem
  Moving 6P Notch Man Z : Subsystem
  Mux : Mux  Inputs=2
  Mux1 : Mux  Inputs=2
  Mx_hat : Outport
  My_hat : Outport  Port=2
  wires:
  omega/1 -> Moving 6P Notch Man Y/2(GenSpeedIN), Moving 3P Notch Man Y/2(GenSpeedIN), Moving 6P Notch Man Z/2(GenSpeedIN), Moving 3P Notch Man Z/2(GenSpeedIN)
  Mx/1 -> Mux/1, Moving 3P Notch Man Y/1(Input)
  My/1 -> Mux1/1, Moving 3P Notch Man Z/1(Input)
  Moving 6P Notch Man Z/1(Output) -> Discrete Filter3/1
  Moving 6P Notch Man Y/1(Output) -> Discrete Filter2/1
  Moving 3P Notch Man Y/1(Output) -> Moving 6P Notch Man Y/1(Input)
  Moving 3P Notch Man Z/1(Output) -> Moving 6P Notch Man Z/1(Input)
  Mux1/1 -> IPC NFs Man 2/2
  Mux/1 -> IPC NFs Man 2/1
  Discrete Filter3/1 -> Mux1/2, My_hat/1
  Discrete Filter2/1 -> Mux/2, Mx_hat/1

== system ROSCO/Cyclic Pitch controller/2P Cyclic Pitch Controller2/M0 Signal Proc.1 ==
  "My1,2, 3" : Inport
  GenSpeed : Inport  Port=2
  Add : Sum  Inputs=+++
  Demux1 : Demux  Outputs=3
  Discrete Filter : DiscreteFilter  Numerator=Parameter.Control.cIPC.PSM0_LPF.Numerator{1}  Denominator=Parameter.Control.cIPC.PSM0_LPF.Denominator{1}  a0EqualsOne=on
  Gain : Gain  Gain=1/3
  Moving 1P Notch Man : Subsystem
  Moving 3P Notch Man : Subsystem
  Mux : Mux  Inputs=2
  Scope : Scope  NumInputPorts=2
  M0 : Outport
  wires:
  Demux1/1 -> Add/1
  Demux1/2 -> Add/2
  Add/1 -> Gain/1
  "My1,2, 3"/1 -> Demux1/1
  GenSpeed/1 -> Moving 3P Notch Man/2(GenSpeedIN), Moving 1P Notch Man/2(GenSpeedIN)
  Demux1/3 -> Add/3
  Moving 1P Notch Man/1(Output) -> Moving 3P Notch Man/1(Input)
  Mux/1 -> Scope/2
  Gain/1 -> Scope/1, Moving 1P Notch Man/1(Input)
  Moving 3P Notch Man/1(Output) -> Discrete Filter/1
  Discrete Filter/1 -> Mux/1, M0/1

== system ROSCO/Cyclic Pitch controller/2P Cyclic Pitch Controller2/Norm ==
  In1 : Inport
  In2 : Inport  Port=2
  Add : Sum
  Discrete Filter1 : DiscreteFilter  Numerator=Parameter.Control.cIPC.IPCDQ_LPF.num{1}  Denominator=Parameter.Control.cIPC.IPCDQ_LPF.den{1}  SampleTime=Parameter.Control.DT
  Product : Product
  Product1 : Product
  Sqrt : Sqrt
  Out1 : Outport
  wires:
  Discrete Filter1/1 -> Out1/1
  In1/1 -> Product/2, Product/1
  In2/1 -> Product1/2, Product1/1
  Add/1 -> Sqrt/1
  Sqrt/1 -> Discrete Filter1/1
  Product1/1 -> Add/2
  Product/1 -> Add/1

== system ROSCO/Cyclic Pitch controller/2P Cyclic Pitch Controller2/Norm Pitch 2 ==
  b_dqsat : Inport
  Demux1 : Demux  Outputs=2
  Sqrt : Sqrt
  Square : Math  Operator=square
  Square1 : Math  Operator=square
  Sum : Sum
  Out1 : Outport
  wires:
  Sqrt/1 -> Out1/1
  Square/1 -> Sum/1
  Demux1/2 -> Square1/1
  Sum/1 -> Sqrt/1
  b_dqsat/1 -> Demux1/1
  Square1/1 -> Sum/2
  Demux1/1 -> Square/1

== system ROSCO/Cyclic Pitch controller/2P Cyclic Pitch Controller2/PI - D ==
  Md : Inport
  Anti-windup : Inport  Port=2
  Discrete Derivative : simulink/Discrete/Discrete Derivative  gainval=1.0  ICPrevScaledInput=0.0  OutMin=[]  OutMax=[]  OutDataType=fixdt(1, 16)  OutScaling=2^-10  DoSatur=off
  Discrete Filter1 : DiscreteFilter  Commented=through  Numerator=Parameter.Control.cIPC.IPCDQ_LPF.num{1}  Denominator=Parameter.Control.cIPC.IPCDQ_LPF.den{1}  SampleTime=Parameter.Control.DT
  Integrator : DiscreteIntegrator  IntegratorMethod=Integration: Backward Euler  gainval=1  SampleTime=simu.dt  UpperSaturationLimit=1.570796/(.008068634/9.5492966)/(1./(1.+pi/2/.109997))  LowerSaturationLimit=0  ICPrevOutput=DiscIntNeverNeededParam  ICPrevScaledInput=DiscIntNeverNeededParam
  Kd : Gain  Gain=0
  Ki : Gain  Gain=R.IPC_KI_2P
  Kp : Gain  Gain=R.IPC_KP_2P
  Sum3 : Sum  Inputs=+++
  Sum8 : Sum  Inputs=|++
  Theta_tilt : Outport
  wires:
  Discrete Filter1/1 -> Kd/1
  Integrator/1 -> Sum3/3
  Discrete Derivative/1 -> Sum3/1
  Kp/1 -> Sum3/2
  Kd/1 -> Discrete Derivative/1
  Sum8/1 -> Integrator/1
  Anti-windup/1 -> Sum8/2
  Md/1 -> Discrete Filter1/1, Kp/1, Ki/1
  Sum3/1 -> Theta_tilt/1
  Ki/1 -> Sum8/1

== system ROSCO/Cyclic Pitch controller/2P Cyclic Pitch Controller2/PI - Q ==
  Mq : Inport
  Anti-windup : Inport  Port=2
  Discrete Derivative : simulink/Discrete/Discrete Derivative  gainval=1.0  ICPrevScaledInput=0.0  OutMin=[]  OutMax=[]  OutDataType=fixdt(1, 16)  OutScaling=2^-10  DoSatur=off
  Discrete Filter1 : DiscreteFilter  Commented=through  Numerator=Parameter.Control.cIPC.IPCDQ_LPF.num{1}  Denominator=Parameter.Control.cIPC.IPCDQ_LPF.den{1}  SampleTime=Parameter.Control.DT
  Integrator1 : DiscreteIntegrator  IntegratorMethod=Integration: Backward Euler  gainval=1  SampleTime=simu.dt  UpperSaturationLimit=1.570796/(.008068634/9.5492966)/(1./(1.+pi/2/.109997))  LowerSaturationLimit=0  ICPrevOutput=DiscIntNeverNeededParam  ICPrevScaledInput=DiscIntNeverNeededParam
  Kd : Gain  Gain=0
  Ki : Gain  Gain=R.IPC_KI_2P
  Kp : Gain  Gain=R.IPC_KP_2P
  Sum10 : Sum  Inputs=|++
  Sum3 : Sum  Inputs=+++
  Theta_yaw : Outport
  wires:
  Discrete Filter1/1 -> Kd/1
  Discrete Derivative/1 -> Sum3/1
  Kd/1 -> Discrete Derivative/1
  Mq/1 -> Ki/1, Kp/1, Discrete Filter1/1
  Kp/1 -> Sum3/2
  Ki/1 -> Sum10/1
  Integrator1/1 -> Sum3/3
  Anti-windup/1 -> Sum10/2
  Sum10/1 -> Integrator1/1
  Sum3/1 -> Theta_yaw/1

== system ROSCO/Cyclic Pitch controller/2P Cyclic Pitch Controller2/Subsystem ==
  Constant3 : Constant  Value=2
  Constant4 : Constant  Value=0
  Constant5 : Constant  Value=0
  Mux : Mux  Inputs=3
  IPC Sat Params : Outport
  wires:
  Constant3/1 -> Mux/1
  Constant4/1 -> Mux/2
  Constant5/1 -> Mux/3
  Mux/1 -> IPC Sat Params/1

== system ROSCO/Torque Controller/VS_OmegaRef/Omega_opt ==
  note: % Assuming known wind speed, initially, and not using GenSpeed
  TSR_opt : Inport
  Wind Speed : Inport  Port=2
  Divide : Product  Inputs=*/
  Multiply : Product
  "Rot -> GenSpeed" : Gain  Gain=R.GBRatio
  Rotor Radius : Constant  Value=R.RotorRad
  Omega_opt : Outport
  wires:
  TSR_opt/1 -> Multiply/1
  Wind Speed/1 -> Multiply/2
  Multiply/1 -> Divide/1
  Rotor Radius/1 -> Divide/2
  Divide/1 -> "Rot -> GenSpeed"/1
  "Rot -> GenSpeed"/1 -> Omega_opt/1

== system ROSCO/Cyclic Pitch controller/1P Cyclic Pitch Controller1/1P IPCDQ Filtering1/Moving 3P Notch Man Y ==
  Input : Inport
  GenSpeedIN : Inport  Port=2
  Gain : Gain  Gain=1/Parameter.Turbine.G * rpm2radps(1) * 3
  Moving 3P Filt Manual : Subsystem
  Slow Low Pass for Param : DiscreteStateSpace  A=Parameter.Control.cIPC.dLPF_slow.a  B=Parameter.Control.cIPC.dLPF_slow.b  C=Parameter.Control.cIPC.dLPF_slow.c  D=Parameter.Control.cIPC.dLPF_slow.d  SampleTime=Parameter.Control.DT
  Output : Outport
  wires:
  Slow Low Pass for Param/1 -> Gain/1
  Gain/1 -> Moving 3P Filt Manual/2(rot speed (rad/s))
  Input/1 -> Moving 3P Filt Manual/1(u)
  GenSpeedIN/1 -> Slow Low Pass for Param/1
  Moving 3P Filt Manual/1(Out1) -> Output/1

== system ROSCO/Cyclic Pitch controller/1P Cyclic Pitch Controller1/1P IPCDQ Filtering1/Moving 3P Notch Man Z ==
  Input : Inport
  GenSpeedIN : Inport  Port=2
  Gain : Gain  Gain=1/Parameter.Turbine.G * rpm2radps(1) * 3
  Moving 3P Filt Manual : Subsystem
  Slow Low Pass for Param : DiscreteStateSpace  A=Parameter.Control.cIPC.dLPF_slow.a  B=Parameter.Control.cIPC.dLPF_slow.b  C=Parameter.Control.cIPC.dLPF_slow.c  D=Parameter.Control.cIPC.dLPF_slow.d  SampleTime=Parameter.Control.DT
  Output : Outport
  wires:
  Moving 3P Filt Manual/1(Out1) -> Output/1
  GenSpeedIN/1 -> Slow Low Pass for Param/1
  Input/1 -> Moving 3P Filt Manual/1(u)
  Gain/1 -> Moving 3P Filt Manual/2(rot speed (rad/s))
  Slow Low Pass for Param/1 -> Gain/1

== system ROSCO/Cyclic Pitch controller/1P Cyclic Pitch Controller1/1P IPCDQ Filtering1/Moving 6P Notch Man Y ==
  Input : Inport
  GenSpeedIN : Inport  Port=2
  Gain : Gain  Gain=1/Parameter.Turbine.G * rpm2radps(1) * 3
  Moving 6P Filt Manual : Subsystem
  Slow Low Pass for Param : DiscreteStateSpace  A=Parameter.Control.cIPC.dLPF_slow.a  B=Parameter.Control.cIPC.dLPF_slow.b  C=Parameter.Control.cIPC.dLPF_slow.c  D=Parameter.Control.cIPC.dLPF_slow.d  SampleTime=Parameter.Control.DT
  Output : Outport
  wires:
  Moving 6P Filt Manual/1(Out1) -> Output/1
  GenSpeedIN/1 -> Slow Low Pass for Param/1
  Input/1 -> Moving 6P Filt Manual/1(u)
  Gain/1 -> Moving 6P Filt Manual/2(rot speed (rad/s))
  Slow Low Pass for Param/1 -> Gain/1

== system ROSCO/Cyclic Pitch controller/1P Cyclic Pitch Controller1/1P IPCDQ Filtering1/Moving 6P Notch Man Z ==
  Input : Inport
  GenSpeedIN : Inport  Port=2
  Gain : Gain  Gain=1/Parameter.Turbine.G * rpm2radps(1) * 3
  Moving 6P Filt Manual : Subsystem
  Slow Low Pass for Param : DiscreteStateSpace  A=Parameter.Control.cIPC.dLPF_slow.a  B=Parameter.Control.cIPC.dLPF_slow.b  C=Parameter.Control.cIPC.dLPF_slow.c  D=Parameter.Control.cIPC.dLPF_slow.d  SampleTime=Parameter.Control.DT
  Output : Outport
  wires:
  Slow Low Pass for Param/1 -> Gain/1
  Gain/1 -> Moving 6P Filt Manual/2(rot speed (rad/s))
  Input/1 -> Moving 6P Filt Manual/1(u)
  GenSpeedIN/1 -> Slow Low Pass for Param/1
  Moving 6P Filt Manual/1(Out1) -> Output/1
